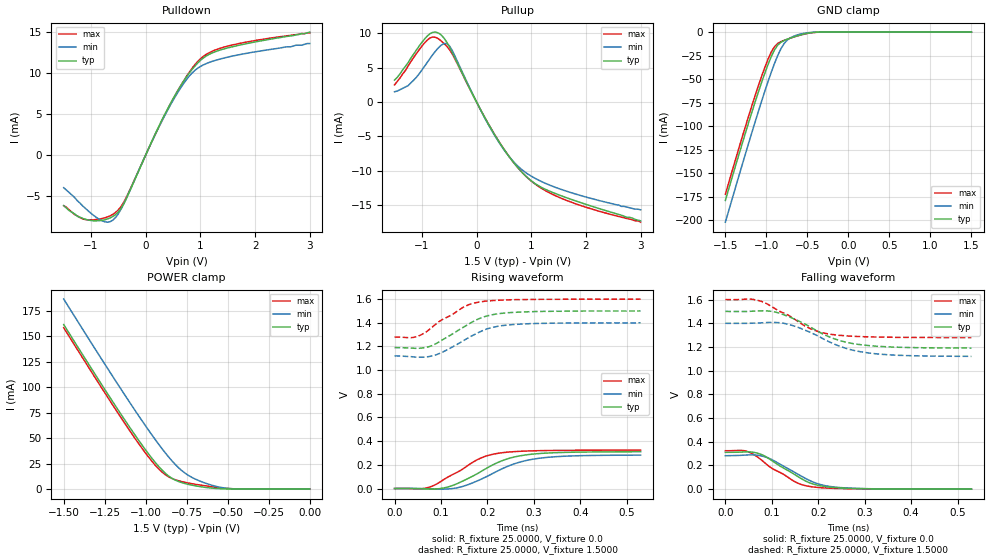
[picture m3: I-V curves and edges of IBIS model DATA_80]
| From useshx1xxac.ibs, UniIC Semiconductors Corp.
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|   Model DATA_80
[Model]  DATA_80
Model_type   I/O
Polarity   Non-Inverting
Enable   Active-High
Vinl =   0.600000V
Vinh =   0.900000V
Vmeas =   0.750000V
Rref =   25.000000
Vref =   0.7500000V
C_comp   1.3900pF   1.3640pF   1.5600pF
[Temperature Range]   25.0000   95.0000   0.0
[Voltage Range]   1.5000V   1.4000V   1.6000V
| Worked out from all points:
|   slope of the pulldown table from 0 to 0.225 V, typ, clamps not added: 68.5 ohm
|   slope of the pullup table from 0 to 0.225 V, typ, clamps not added: 67.8 ohm
|   GND clamp passes 1 mA (typ) near -0.48 V on its own axis
|   POWER clamp passes 1 mA (typ) near -0.59 V on its own axis
|   rising waveform, R_fixture 25.0000, V_fixture 0.0: 20-80 % time 95.2ps typ, 98.9ps min, 85.4ps max; typ from 0 V to 0.311 V
|   rising waveform, R_fixture 25.0000, V_fixture 1.5000: 20-80 % time 82.7ps typ, 80.9ps min, 75.4ps max; typ from 1.19 V to 1.5 V
|   falling waveform, R_fixture 25.0000, V_fixture 0.0: 20-80 % time 79.2ps typ, 80.1ps min, 75.5ps max; typ from 0.311 V to 0 V
|   falling waveform, R_fixture 25.0000, V_fixture 1.5000: 20-80 % time 101ps typ, 101ps min, 88.1ps max; typ from 1.5 V to 1.19 V
[Pulldown]
|Voltage   I(typ)   I(min)   I(max)
-1.5V     -6.2mA     -4mA       -6.2mA
-1.1V     -7.87mA    -6.55mA    -7.9mA
-800mV    -7.989mA   -8.05mA    -7.772mA
-600mV    -7.517mA   -7.961mA   -7.253mA
-400mV    -5.963mA   -5.942mA   -5.76mA
100mV     1.497mA    1.449mA    1.455mA
450mV     6.253mA    6.074mA    6.179mA
700mV     9.07mA     8.787mA    9.107mA
900mV     10.85mA    10.33mA    11.03mA
1.15V     12.25mA    11.27mA    12.44mA
1.45V     12.98mA    11.86mA    13.2mA
3V        15mA       13.6mA     14.9mA
[Pullup]
|Voltage   I(typ)   I(min)   I(max)
-1.5V     3.2mA      1.5mA      2.5mA
-1.25V    5.77mA     2.4mA      5.28mA
-850mV    9.96mA     6.36mA     9.34mA
-700mV    10.06mA    7.88mA     9.228mA
-550mV    8.786mA    8.526mA    8.173mA
-450mV    7.293mA    7.583mA    7.068mA
300mV     -4.346mA   -4.459mA   -4.329mA
550mV     -7.444mA   -7.477mA   -7.431mA
800mV     -9.959mA   -9.656mA   -9.97mA
1.1V      -12.03mA   -11.24mA   -12.11mA
1.5V      -13.51mA   -12.59mA   -13.85mA
3V        -17.3mA    -15.7mA    -17.5mA
[GND_clamp]
|Voltage   I(typ)   I(min)   I(max)
-1.5V     -178.7mA   -201.8mA   -172.1mA
-1.18V    -85.9mA    -107.5mA   -79.02mA
-1.06V    -53.85mA   -73.82mA   -47.38mA
-980mV    -34.46mA   -52.52mA   -28.79mA
-940mV    -25.94mA   -42.47mA   -21.09mA
-900mV    -18.8mA    -33.04mA   -15.34mA
-860mV    -13.68mA   -24.5mA    -11.91mA
-780mV    -8.804mA   -11.75mA   -8.617mA
-740mV    -7.413mA   -8.071mA   -7.384mA
-620mV    -3.934mA   -2.917mA   -4.046mA
-420mV    -302.4uA   -187.9uA   -428.5uA
1.5V      1.623nA    17.64nA    1.98nA
[POWER_clamp]
|Voltage   I(typ)   I(min)   I(max)
-1.5V     161.3mA    186.3mA    158.3mA
-1.22V    90.37mA    115.2mA    87.1mA
-1.04V    47.2mA     71.18mA    43.94mA
-980mV    33.96mA    57.17mA    30.91mA
-920mV    22.07mA    43.79mA    19.67mA
-880mV    15.49mA    35.42mA    14.07mA
-840mV    10.61mA    27.72mA    10.46mA
-780mV    6.409mA    18.15mA    7.405mA
-720mV    3.991mA    11.66mA    5.381mA
-560mV    586.1uA    2.318mA    1.645mA
-440mV    47uA       184.9uA    218uA
0V        1.623nA    5.301nA    2.263nA
[Ramp]
| variable   typ   min   max
dV/dt_r  0.1867/96.3613p   0.1696/99.8013p   0.1946/86.0717p
dV/dt_f  0.1860/0.1017n   0.1680/0.1020n   0.1926/88.8214p
R_load = 25.0000
[Rising Waveform]
R_fixture= 25.0000
V_fixture= 0.0
V_fixture_min= 0.0
V_fixture_max= 0.0
|time   V(typ)   V(min)   V(max)
0s        0V         0V         0V
65ps      -2.457mV   -1.226mV   1.958mV
85ps      -4.334mV   -3.958mV   26.66mV
115ps     13.26mV    -3.416mV   97.12mV
145ps     59.68mV    15.91mV    160.1mV
180ps     129.4mV    67.64mV    246.9mV
225ps     224.4mV    154.3mV    298.7mV
270ps     276mV      223.3mV    314.4mV
320ps     297.8mV    259.7mV    320.3mV
530ps     310.6mV    282.1mV    324.3mV
[Rising Waveform]
R_fixture= 25.0000
V_fixture= 1.5000
V_fixture_min= 1.4000
V_fixture_max= 1.6000
|time   V(typ)   V(min)   V(max)
0s        1.19V      1.12V      1.279V
45ps      1.184V     1.11V      1.28V
60ps      1.187V     1.109V     1.304V
75ps      1.199V     1.115V     1.343V
105ps     1.26V      1.155V     1.431V
150ps     1.366V     1.252V     1.535V
185ps     1.439V     1.325V     1.577V
210ps     1.467V     1.36V      1.587V
255ps     1.487V     1.385V     1.594V
530ps     1.5V       1.4V       1.6V
[Falling Waveform]
R_fixture= 25.0000
V_fixture= 0.0
V_fixture_min= 0.0
V_fixture_max= 0.0
|time   V(typ)   V(min)   V(max)
0s        310.6mV    282.1mV    324.3mV
45ps      314.6mV    288mV      320.7mV
75ps      296.2mV    282.6mV    254.7mV
100ps     241.2mV    249.5mV    176.4mV
150ps     121.5mV    140.1mV    62.27mV
165ps     85.44mV    106.9mV    37.66mV
185ps     48.47mV    66.79mV    20.79mV
215ps     21.84mV    29.56mV    9.999mV
265ps     7.342mV    9.215mV    3.74mV
530ps     0V         0V         0V
[Falling Waveform]
R_fixture= 25.0000
V_fixture= 1.5000
V_fixture_min= 1.4000
V_fixture_max= 1.6000
|time   V(typ)   V(min)   V(max)
0s        1.5V       1.4V       1.6V
60ps      1.502V     1.401V     1.601V
85ps      1.505V     1.405V     1.573V
110ps     1.492V     1.406V     1.516V
140ps     1.45V      1.386V     1.458V
175ps     1.386V     1.336V     1.369V
220ps     1.291V     1.25V      1.311V
265ps     1.236V     1.182V     1.292V
310ps     1.211V     1.148V     1.285V
530ps     1.19V      1.12V      1.279V
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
